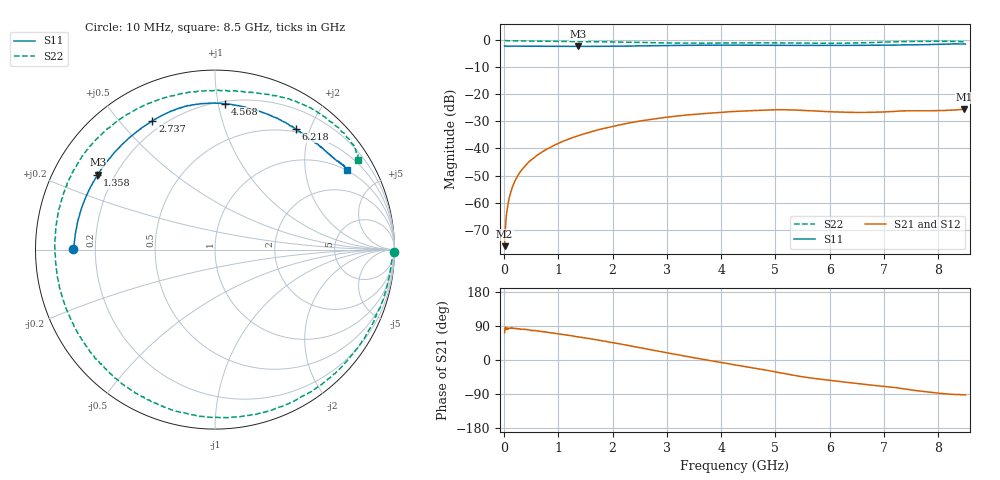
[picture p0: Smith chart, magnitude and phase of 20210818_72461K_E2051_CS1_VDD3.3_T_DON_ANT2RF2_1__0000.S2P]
!Agilent Technologies,E5071C,MY46417908,A.11.23
!Date: Wed Aug 18 14:26:03 2021
!Data & Calibration Information:
!Freq	S11:SOLT2(ON)	S21:SOLT2(ON)	S12:SOLT2(ON)	S22:SOLT2(ON)
!PortZ  Port1:50+j0  Port2:50+j0
!Above PortZ is port z conversion or system Z0 setting when saving the data.
!When reading, reference impedance value at option line is always used.
# Hz S dB R 50
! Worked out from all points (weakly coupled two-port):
!   1601 points, 10 MHz to 8.5 GHz, reference 50 ohm
!   highest |S21| = -25.49 dB at 8.479 GHz (marker M1); lowest = -76.1 dB at 10 MHz (marker M2)
!   lowest |S11| = -2.2 dB at 1.368 GHz (marker M3), VSWR 7.86, Z = 6.9 + j14.4 ohm
!   |S11| at or under -10 dB: nowhere
!   |S22| runs from -1.1 to 0.0 dB; largest |S21 - S12| = 0.00028
!   S11 on the Smith chart (normalised r, x): 10 MHz: 0.12, +0.00; 1.358 GHz: 0.14, +0.29; 2.737 GHz: 0.16, +0.61; 4.568 GHz: 0.22, +1.05; 6.218 GHz: 0.46, +1.78; 8.5 GHz: 1.00, +3.34
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1e7  -2.06 179.7  -76.15 72.1  -75.79 84.7  -0.01 -0.6
6.836875e7  -2.10 178.4  -61.11 83.0  -61.26 81.1  -0.11 -3.3
1.108188e8  -2.10 177.4  -57.03 83.9  -57.02 83.8  -0.13 -5.2
1.904125e8  -2.12 175.6  -52.42 83.6  -52.44 83.8  -0.16 -8.5
3.0715e8  -2.14 172.9  -48.40 81.3  -48.40 81.6  -0.19 -13.6
7.3165e8  -2.18 162.9  -40.91 74.6  -40.90 74.7  -0.29 -31.5
1.357788e9  -2.21 147.6  -35.33 61.1  -35.33 61.2  -0.43 -58.6
1.3684e9  -2.22 147.4  -35.27 60.8  -35.28 60.9  -0.44 -59.0
1.426769e9  -2.21 145.8  -34.88 59.7  -34.89 59.5  -0.43 -61.6
2.116581e9  -2.13 128.9  -31.31 42.9  -31.31 42.9  -0.61 -93.3
2.737412e9  -1.96 115.9  -29.10 26.1  -29.09 26.2  -0.82 -124.8
2.843538e9  -1.94 114.1  -28.81 23.2  -28.82 23.2  -0.87 -130.5
3.517431e9  -1.80 103.4  -27.36 5.5  -27.37 5.5  -1.00 -166.0
4.255e9  -1.76 91.7  -26.29 -12.9  -26.29 -12.8  -0.91 158.5
4.568069e9  -1.79 86.2  -25.99 -20.5  -26.00 -20.5  -0.87 144.9
5.178288e9  -1.83 74.1  -25.66 -36.3  -25.67 -36.2  -0.96 120.2
5.671769e9  -1.84 64.8  -26.07 -47.8  -26.05 -47.7  -1.02 102.4
6.218312e9  -1.86 56.1  -26.53 -57.2  -26.53 -57.3  -1.04 86.0
7.088538e9  -1.72 45.0  -26.38 -71.0  -26.42 -71.2  -0.57 63.2
7.916312e9  -1.48 35.7  -26.02 -86.0  -25.99 -86.0  -0.28 42.0
8.478775e9  -1.31 31.0  -25.49 -91.9  -25.50 -91.9  -0.50 32.4
8.5e9  -1.33 30.9  -25.50 -91.9  -25.51 -92.0  -0.55 32.0
